FUNCTION FC 70 : VOID
TITLE =BLOCK FOR LUBRICATION
AUTHOR : Esposito
FAMILY : EGAL_srl
NAME : LUBRIFIC
VERSION : 0.1

BEGIN
NETWORK
TITLE =CONDITIONS FOR START PUMP LUBRICATION
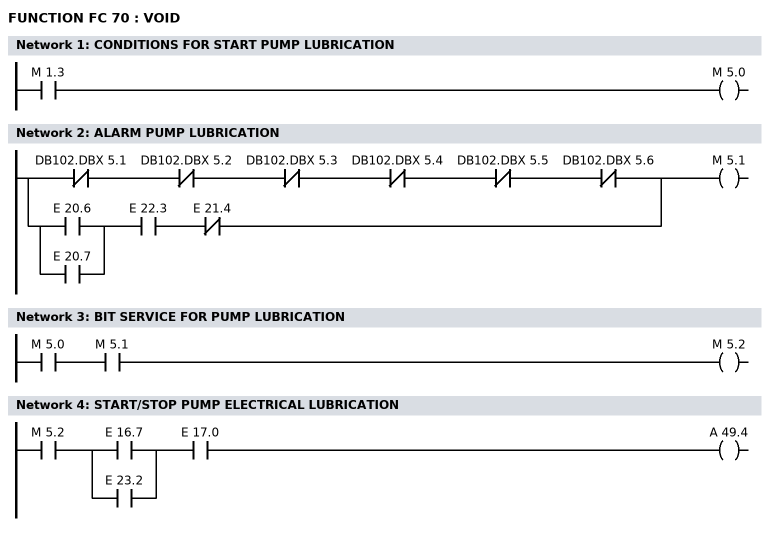
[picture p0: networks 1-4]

      U     M      1.3;
      =     M      5.0;
NETWORK
TITLE =ALARM PUMP LUBRICATION

      UN    DB102.DBX    5.1;
      UN    DB102.DBX    5.2;
      UN    DB102.DBX    5.3;
      UN    DB102.DBX    5.4;
      UN    DB102.DBX    5.5;
      UN    DB102.DBX    5.6;
      O     ;
      U(    ;
      O     E     20.6;
      O     E     20.7;
      )     ;
      U     E     22.3;
      UN    E     21.4;
      =     M      5.1;
NETWORK
TITLE =BIT SERVICE FOR PUMP LUBRICATION

      U     M      5.0;
      U     M      5.1;
      =     M      5.2;
NETWORK
TITLE =START/STOP PUMP ELECTRICAL LUBRICATION

      U     M      5.2;
      U(    ;
      O     E     16.7;
      O     E     23.2;
      )     ;
      U     E     17.0;
      =     A     49.4;
NETWORK
TITLE =TIME PAUSE AND JOB TRABON

      L     DB15.DBW   82;
      ITB   ;
      L     W#16#3000;
      OW    ;
      T     MW    50;
//;
      L     DB15.DBW   84;
      ITB   ;
      L     W#16#3000;
      OW    ;
      T     MW    52;
NETWORK
TITLE =TIMER PAUSE AND JOB PUMP LUBRICATION TRABON
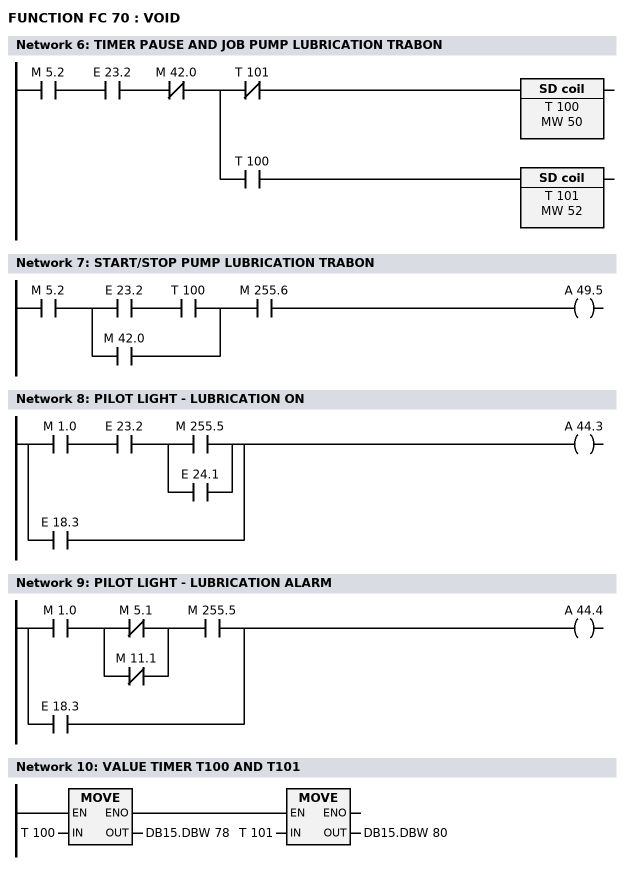
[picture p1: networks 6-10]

      U     M      5.2;
      U     E     23.2;
      UN    M     42.0;
      =     L      0.0;
      U     L      0.0;
      UN    T    101;
      L     MW    50;
      SE    T    100;
      U     L      0.0;
      U     T    100;
      L     MW    52;
      SE    T    101;
NETWORK
TITLE =START/STOP PUMP LUBRICATION TRABON

      U     M      5.2;
      U(    ;
      U     E     23.2;
      U     T    100;
      O     M     42.0;
      )     ;
      U     M    255.6;
      =     A     49.5;
NETWORK
TITLE =PILOT LIGHT - LUBRICATION ON

      U     M      1.0;
      U     E     23.2;
      U(    ;
      O     M    255.5;
      O     E     24.1;
      )     ;
      O     E     18.3;
      =     A     44.3;
NETWORK
TITLE =PILOT LIGHT - LUBRICATION ALARM

      U     M      1.0;
      U(    ;
      ON    M      5.1;
      ON    M     11.1;
      )     ;
      U     M    255.5;
      O     E     18.3;
      =     A     44.4;
NETWORK
TITLE =VALUE TIMER T100 AND T101

      L     T    100;
      T     DB15.DBW   78;
//;
      L     T    101;
      T     DB15.DBW   80;

END_FUNCTION

